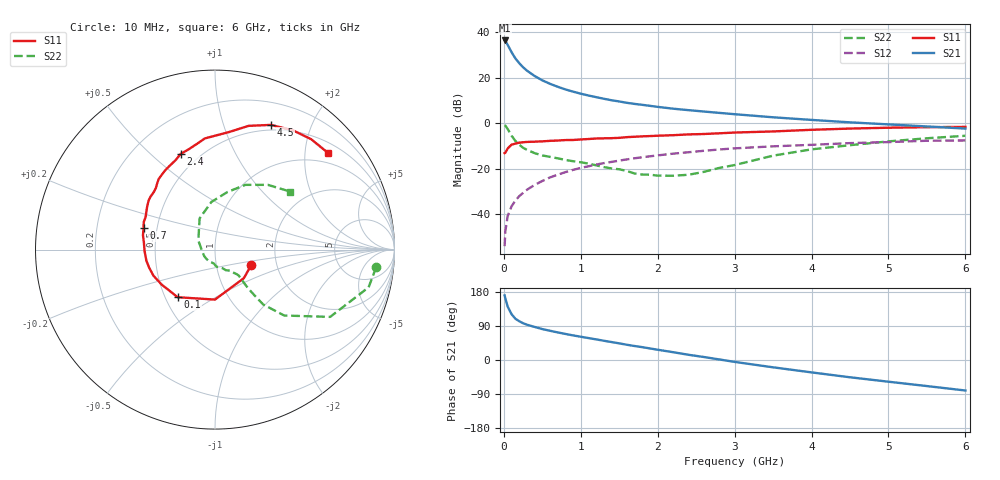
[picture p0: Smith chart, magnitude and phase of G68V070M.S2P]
! SIEMENS Small Signal Semiconductors
! BFG193
! Si NPN RF Bipolar Junction Transistor in SOT223
! VCE = 8 V  IC = 70 mA
! Common Emitter S-Parameters:  August  1996
# GHz  S  MA  R  50
!  f  S11  S21  S12  S22
! GHz  MAG  ANG  MAG  ANG  MAG  ANG  MAG  ANG
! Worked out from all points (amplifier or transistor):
!   36 points, 10 MHz to 6 GHz, reference 50 ohm
!   highest |S21| = 36.3 dB at 10 MHz (marker M1)
!   |S21| within 3 dB of that: start of sweep to 66.61 MHz
!   unconditionally stable (mu >= 1): 392.7 MHz to 2.377 GHz
!   at 250 MHz: K = 0.94, MSG = 27.6 dB, |S12| = -30.6 dB
!   at 1.4 GHz: K = 1.05, MAG = 12.2 dB, |S12| = -17.0 dB
!   at 6 GHz: K = 0.89, MSG = 2.6 dB, |S12| = -7.6 dB
!   S11 on the Smith chart (normalised r, x): 10 MHz: 1.48, -0.27; 100 MHz: 0.58, -0.35; 700 MHz: 0.42, +0.12; 2.4 GHz: 0.40, +0.63; 4.5 GHz: 0.44, +1.45; 6 GHz: 0.73, +2.52
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0.01  0.22 -22.9  65.22 170.3  0.002 84.4  0.903 -6.3
0.02  0.2263 -44.9  62.53 162.3  0.0043 78.6  0.8812 -13.8
0.05  0.2784 -90.0  52.12 140.8  0.0092 72.4  0.7432 -30.3
0.1  0.3372 -128.1  36.2 121.0  0.0149 67.9  0.5327 -43.6
0.15  0.356 -147.1  26.35 108.9  0.0201 67.8  0.4072 -48.7
0.2  0.3726 -157.1  20.71 102.3  0.025 69.2  0.3386 -49.2
0.25  0.3807 -164.9  16.86 97.1  0.0295 70.2  0.288 -49.4
0.3  0.3873 -170.9  14.22 93.1  0.0346 70.5  0.2602 -49.2
0.4  0.3923 -178.7  10.83 87.3  0.0441 70.2  0.2199 -48.2
0.5  0.3988 173.8  8.702 81.6  0.0539 69.6  0.1959 -47.6
0.6  0.4091 168.9  7.301 77.2  0.0644 68.6  0.1821 -48.6
0.7  0.4153 163.4  6.29 72.8  0.0741 67.2  0.1695 -50.6
0.9  0.4271 154.8  4.915 64.9  0.0944 63.3  0.1461 -53.7
1.1  0.4488 147.2  4.041 57.9  0.1132 59.9  0.1297 -62.3
1.3  0.4646 140.8  3.429 50.8  0.1328 55.8  0.1087 -69.6
1.6  0.4937 130.4  2.794 40.2  0.1602 49.1  0.0891 -88.4
2.2  0.5443 113.8  2.078 20.6  0.2141 35.5  0.0702 -148.4
2.4  0.5665 109.7  1.929 13.8  0.2301 31.3  0.0737 -177.2
3.5  0.6581 83.5  1.345 -19.3  0.3099 4.3  0.1937 116.3
4.5  0.761 65.9  1.042 -45.6  0.3649 -15.7  0.3283 77.8
5.5  0.8156 48.9  0.847 -68.8  0.4113 -39.2  0.4661 50.7
6  0.8286 40.6  0.76 -80.5  0.4173 -52.6  0.5287 37.7
